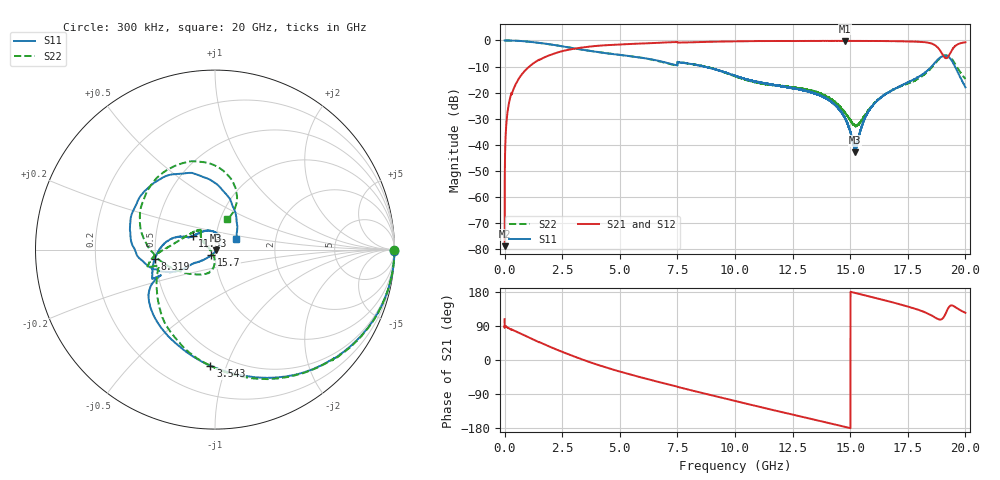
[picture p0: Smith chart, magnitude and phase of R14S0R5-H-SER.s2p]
!{R14S0R5}
!Johanson Technology Inc.
!www.johansontechnology.com
!Test Board Conditions:
!Substrate Type  RO4350B
!Substrate Thickness  20 mil
!Substrate Dk  3.66
!TL Type: GCPW
!TL Trace Width  36 mil
!TL Gap  12 mil
!Electrode orientation  Horizontal
!DUT TOPOLOGY	SERIES
!Mounting Pad LxW  26x36 mil
! Created Wed Nov 25 17:33:21 2020
! 2 Port Network Data from SP1.SP block
! freq  magS11  angS11  magS21  angS21  magS12  angS12  magS22  angS22
# khz S ma R 50
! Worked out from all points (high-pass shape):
!   20001 points, 300 kHz to 20 GHz, reference 50 ohm
!   highest |S21| = -0.15 dB at 14.79 GHz (marker M1); lowest = -78.7 dB at 300 kHz (marker M2)
!   |S21| within 3 dB of the highest: 3.036 GHz to 18.84 GHz (15.81 GHz wide, 144 % of centre); 19.45 GHz to end of sweep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
!   lowest |S11| = -42.7 dB at 15.22 GHz (marker M3), VSWR 1.01, Z = 50.6 - j0.462 ohm
!   |S11| at or under -10 dB: 8.661952 GHz to 8.664223 GHz (2.271 MHz wide, 0.0262 % of centre); 8.667 GHz to 18.53 GHz (9.861 GHz wide, 72.5 % of centre); 19.55 GHz to end of sweep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
!   |S22| runs from -32.9 to 0.0 dB; largest |S21 - S12| = 0.013
!   S11 on the Smith chart (normalised r, x): 300 kHz: open; 3.543 GHz: 0.39, -0.88; 8.319 GHz: 0.50, -0.06; 11.53 GHz: 0.77, +0.12; 15.7 GHz: 0.96, -0.06; 20 GHz: 1.25, +0.14
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300  0.9978 -0.4  0.0001157 107.8  7.645e-05 109.9  0.9983 -0.2
101300  0.9991 -3.2  0.03377 86.5  0.03406 86.5  0.9993 -3.3
134300  0.9985 -4.2  0.04484 85.5  0.04494 85.5  0.9989 -4.2
512300  0.9871 -14.7  0.155 74.8  0.1552 74.9  0.9864 -14.8
1857300  0.8566 -51.5  0.5025 37.8  0.5035 37.9  0.8552 -52.2
3334300  0.6692 -87.5  0.7295 2.2  0.7299 2.2  0.6703 -87.9
3543300  0.6478 -92.3  0.7491 -2.4  0.7503 -2.4  0.648 -92.2
5120300  0.5217 -126.8  0.8416 -32.7  0.8419 -32.6  0.5219 -118.0
6667300  0.4089 -150.7  0.9019 -57.6  0.9035 -57.5  0.4033 -143.3
8319300  0.3397 -170.9  0.9276 -83.3  0.9295 -83.1  0.342 -173.5
1.00003e7  0.2125 159.9  0.9629 -108.1  0.9655 -108.1  0.2066 165.8
1.15253e7  0.1447 149.0  0.9753 -130.3  0.9767 -130.3  0.1417 130.7
1.33343e7  0.09994 94.4  0.9787 -155.8  0.9775 -155.8  0.1093 136.4
1.47903e7  0.0322 42.4  0.9828 -176.8  0.9804 -176.7  0.04079 160.9
1.52243e7  0.007289 -38.8  0.9786 176.9  0.9816 176.9  0.02367 -153.7
1.56983e7  0.03662 -123.8  0.979 169.7  0.9778 169.7  0.04129 -98.8
1.66673e7  0.1014 -141.9  0.972 154.8  0.9684 154.9  0.1025 -95.8
1.84303e7  0.2853 -153.9  0.8969 120.8  0.8919 120.8  0.2708 -159.1
1.88543e7  0.4522 178.7  0.6867 107.0  0.6897 106.7  0.4413 161.2
1.90983e7  0.5091 147.7  0.4771 116.7  0.4783 116.6  0.5158 127.4
1.94993e7  0.3488 85.3  0.7369 141.9  0.7437 141.9  0.3899 75.2
2e7  0.1272 25.7  0.9242 124.6  0.9221 124.7  0.1835 68.4
